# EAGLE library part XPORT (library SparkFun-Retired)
TCP/IP stack and phy in RJ-45 jack footprint
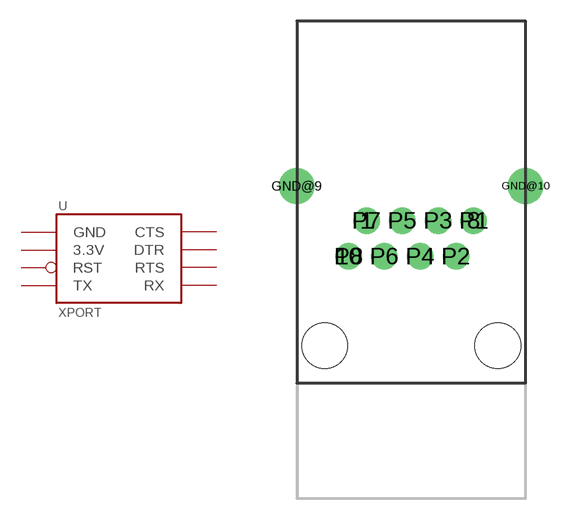
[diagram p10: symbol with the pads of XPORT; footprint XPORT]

Designator prefix -

## XPORT  [XPORT]
P1  GND
P2  3.3V
P3  RST
P4  TX
P5  RX
P6  RTS
P7  DTR
P8  CTS

## Footprint XPORT (pad centres in mm)
drill 0.889 pad 1.88: 1 -3.175,7.62; 8 4.445,7.62; 10 -4.445,5.08; P1 4.445,7.62; P2 3.175,5.08; P3 1.905,7.62; P4 0.635,5.08; P5 -0.635,7.62; P6 -1.905,5.08; P7 -3.175,7.62; P8 -4.445,5.08
drill 1.6 pad 2.54: GND@9 -8.128,10.081; GND@10 8.128,10.081
hole 3.251 at -6.147,-1.27
hole 3.251 at 6.147,-1.27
